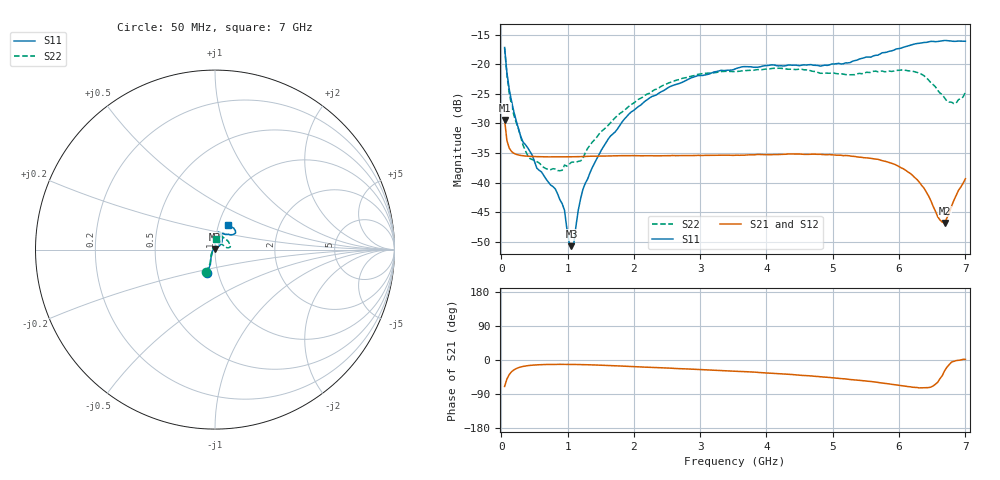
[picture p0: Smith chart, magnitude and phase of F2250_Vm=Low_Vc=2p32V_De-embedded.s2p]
! Integrated Device Technology
! Corporate Headquarters
! 6024 Silver Creek Valley Road
! San Jose, CA 95138  USA
! Phone:  1-408-284-8200
! Toll Free:  1-800-223-1366
! Webpage:  http://www.idt.com/
! Timing and RF Division
! 515 Groton Road, Suite 102
! Westford, MA 01886-6024
! Device:  F2250
! Description: Voltage Variable RF Attenuator
! Frequency:  50.0 -  6000.00 MHz
! Package:  3x3 mm Thin QFN Plastic Package: 16 pin
! Ports:  2 RF, 3 DC
!  Pin  1  = GND
!  Pin  2  = NC
!  Pin  3  = RF1  = Port 1
!  Pin  4  = NC
!  Pin  5  = GND
!  Pin  6  = GND
!  Pin  7  = GND
!  Pin  8  = GND
!  Pin  9  = NC
!  Pin 10  = RF2  = Port 2
!  Pin 11  = NC
!  Pin 12  = GND
!  Pin 13  = GND
!  Pin 14  = VCNTRL
!  Pin 15  = VDD
!  Pin 16  = VMODE
! Vcntrl:  2.320 Volts
! Vmode:  +0.000 Volts
! Vdd:  +3.30  Volts
! Current:  1.177 mA
! Data:  The device was measured on a the F2250 evaluation board which has
!  individual transmission lines to the RF pins.  Data was collected
!  using a calibrated network analyzer.  The evaluation board was
!  de-embedded using a TRL calibration technique.
!  The reference plane is the edge of the package pin.
! Misc:  SN 10
!  Action Tracker AT0258
! Date Measured:  2014-11-26
! Date:  2015-10-15  MJV
! Note:
!  Integrated Device Technology supplies this data as a sample of measured
!  data at the package pin for this product.  Your particular data for this
!  product may vary.
!  Data was taken at 25 degrees C.
!  Integrated Device Technology reserves the right to change this data at anytime.
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# GHz S dB R 50
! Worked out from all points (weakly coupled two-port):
!   201 points, 50 MHz to 7 GHz, reference 50 ohm
!   highest |S21| = -29.40 dB at 50 MHz (marker M1); lowest = -46.8 dB at 6.687 GHz (marker M2)
!   lowest |S11| = -50.7 dB at 1.058 GHz (marker M3), VSWR 1.01, Z = 49.8 + j0.244 ohm
!   |S11| at or under -10 dB: start of sweep to end of sweep
!   |S22| runs from -38.0 to -17.3 dB; largest |S21 - S12| = 5.6e-05
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0.05  -17.18 -108.7  -29.40 -69.7  -29.40 -69.7  -17.31 -110.9
0.08475  -21.44 -107.4  -32.90 -50.3  -32.90 -50.3  -21.80 -109.8
0.15425  -26.23 -116.6  -34.73 -31.1  -34.73 -31.1  -26.91 -121.7
0.29325  -32.20 -127.7  -35.41 -18.4  -35.41 -18.4  -32.30 -136.4
0.3975  -34.09 -141.8  -35.54 -15.0  -35.54 -15.0  -35.39 -159.6
0.91875  -43.56 158.2  -35.66 -11.5  -35.66 -11.5  -37.91 131.5
0.9535  -44.67 169.5  -35.66 -11.5  -35.65 -11.5  -37.02 129.6
1.023  -50.10 144.2  -35.65 -11.6  -35.65 -11.6  -36.90 113.8
1.05775  -50.73 122.7  -35.64 -11.6  -35.64 -11.6  -36.55 108.6
1.0925  -50.38 90.3  -35.63 -11.7  -35.63 -11.7  -36.52 103.8
1.162  -44.59 57.0  -35.61 -11.9  -35.61 -11.9  -36.40 92.9
1.2315  -41.13 44.2  -35.58 -12.1  -35.59 -12.1  -35.89 83.4
1.6485  -32.12 41.9  -35.50 -14.7  -35.49 -14.7  -29.88 63.3
1.9265  -28.40 41.3  -35.44 -16.9  -35.44 -16.9  -27.09 55.8
2.37825  -24.87 47.4  -35.46 -20.3  -35.45 -20.3  -24.00 56.2
3.525  -20.80 72.5  -35.38 -29.6  -35.38 -29.6  -21.24 74.5
4.7065  -20.17 72.3  -35.18 -42.6  -35.18 -42.6  -21.21 72.1
5.85325  -17.81 40.5  -36.61 -63.3  -36.62 -63.3  -21.17 22.6
6.27025  -16.50 40.1  -39.47 -72.6  -39.47 -72.7  -21.38 9.3
6.68725  -15.99 48.8  -46.81 -28.2  -46.77 -27.8  -25.71 28.1
6.861  -16.13 55.1  -42.17 -1.5  -42.13 -1.6  -26.56 58.0
7  -16.12 63.2  -39.34 1.6  -39.30 1.5  -24.69 83.3
